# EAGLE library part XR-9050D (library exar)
Data SYNCHRONIZER/RLL ENDEC
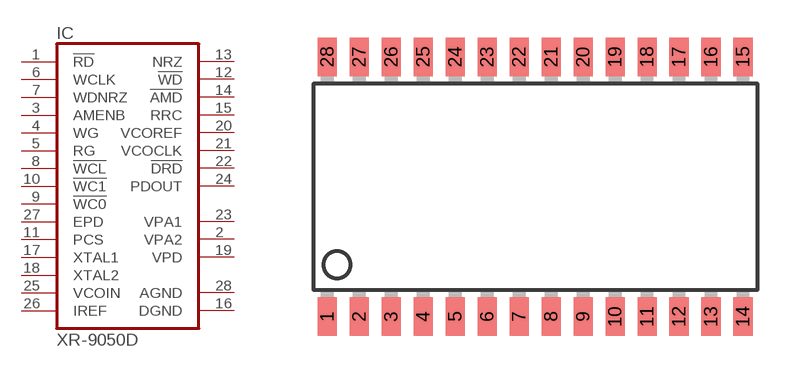
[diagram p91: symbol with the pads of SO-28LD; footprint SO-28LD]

Designator prefix IC

## XR-9050D (OC_FARNELL: unknown; OC_NEWARK: unknown)  [SO-28LD]
1  !RD  in
2  VPA2  pwr
3  AMENB  in
4  WG  in
5  RG  in
6  WCLK  in
7  WDNRZ  in
8  !WCL  in
9  !WC0  in
10  !WC1  in
11  PCS  in
12  !WD  out
13  NRZ
14  !AMD  out
15  RRC  out
16  DGND  pwr
17  XTAL1  in
18  XTAL2  in
19  VPD  pwr
20  VCOREF  out
21  VCOCLK  out
22  !DRD  out
23  VPA1  pwr
24  PDOUT  out
25  VCOIN  in
26  IREF  in
27  EPD  in
28  AGND  pwr

## Footprint SO-28LD (pad centres in mm)
Small Outline Package
smd 0.762 x 1.524: 1 -8.255,-5.156; 2 -6.985,-5.156; 3 -5.715,-5.156; 4 -4.445,-5.156; 5 -3.175,-5.156; 6 -1.905,-5.156; 7 -0.635,-5.156; 8 0.635,-5.156; 9 1.905,-5.156; 10 3.175,-5.156; 11 4.445,-5.156; 12 5.715,-5.156; 13 6.985,-5.156; 14 8.255,-5.156; 15 8.255,5.156; 16 6.985,5.156; 17 5.715,5.156; 18 4.445,5.156; 19 3.175,5.156; 20 1.905,5.156; 21 0.635,5.156; 22 -0.635,5.156; 23 -1.905,5.156; 24 -3.175,5.156; 25 -4.445,5.156; 26 -5.715,5.156; 27 -6.985,5.156; 28 -8.255,5.156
